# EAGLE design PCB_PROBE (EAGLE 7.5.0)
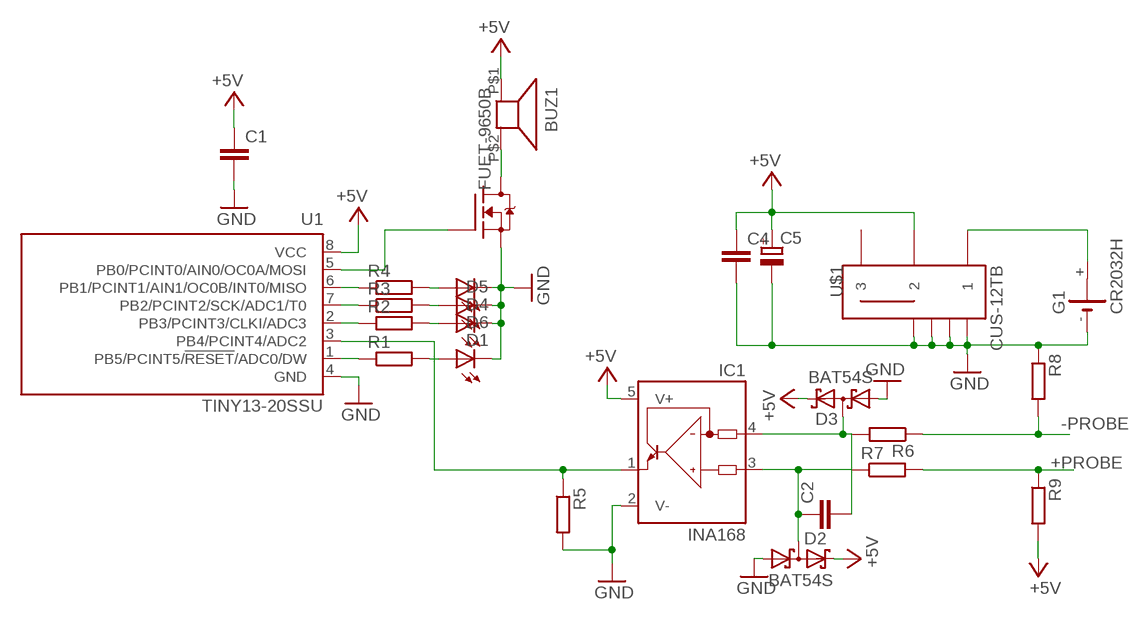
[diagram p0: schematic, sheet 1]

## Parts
BUZ1  FUET-9650B  [FUET-9650B]
C1  C-EUC0603  [C0603]
C2  C-EUC0603  [C0603]
C4  C-EUC0603  [C0603]
C5  CPOL-EUSMCC  [SMC_C]
D1  LEDCHIPLED_0805  [CHIPLED_0805]
D2  BAT54S  [SOT23]
D3  BAT54S  [SOT23]
D4  LEDCHIPLED_0805  [CHIPLED_0805]
D5  LEDCHIPLED_0805  [CHIPLED_0805]
D6  LEDCHIPLED_0805  [CHIPLED_0805]
G1  CR2032H  [CR2032H]
IC1  INA168  [SOT23-5]
Q1  ZVN3310F  [SOT23]
R1  R-EU_R0603  [R0603]
R2  R-EU_R0603  [R0603]
R3  R-EU_R0603  [R0603]
R4  R-EU_R0603  [R0603]
R5  R-EU_R0603  [R0603]
R6  R-EU_R0603  [R0603]
R7  R-EU_R0603  [R0603]
R8  R-EU_R0603  [R0603]
R9  R-EU_R0603  [R0603]
U1  TINY13-20SSU  [8S1]
U$1  CUS-12TB  [CUS-12B]

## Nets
+5V: BUZ1.P$1 C1.1 C4.1 C5.+ D2.2(C2) D3.2(C2) IC1.5(V+) R9.2 U1.8(VCC) U$1.P$2
+PROBE: R7.2 R9.1
-PROBE: R6.1 R8.2
GND: C1.2 C4.2 C5.- D1.C D2.1(A1) D3.1(A1) D4.C D5.C D6.C G1.- IC1.2(V-) Q1.3(S) R5.2 R8.1 U1.4(GND) U$1.P$4(GND) U$1.P$5(GND) U$1.P$6(GND) U$1.P$7(GND)
N$1: G1.+ U$1.P$1
N$2: R1.1 U1.1(PB5/PCINT5/!RESET!/ADC0/DW)
N$3: R2.1 U1.2(PB3/PCINT3/CLKI/ADC3)
N$4: R3.1 U1.7(PB2/PCINT2/SCK/ADC1/T0)
N$5: R4.1 U1.6(PB1/PCINT1/AIN1/OC0B/INT0/MISO)
N$6: D6.A R4.2
N$7: D5.A R3.2
N$8: D4.A R2.2
N$9: D1.A R1.2
N$10: IC1.1(OUT) R5.1 U1.3(PB4/PCINT4/ADC2)
N$11: C2.2 D3.3(C1A2) IC1.4(IN-) R6.2
N$12: C2.1 D2.3(C1A2) IC1.3(IN+) R7.1
N$13: Q1.2(G) U1.5(PB0/PCINT0/AIN0/OC0A/MOSI)
N$14: BUZ1.P$2 Q1.1(D)
Unconnected: G1.+@1(+) U$1.P$3

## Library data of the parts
BUZ1 = buzzer:FUET-9650B
C1 C2 C4 = rcl:C-EU: CAPACITOR, European symbol
C5 = rcl:CPOL-EU: POLARIZED CAPACITOR, European symbol
D1 D4-D6 = led:LED: LED
D2 D3 = diode:BAT54S: Schottky Diodes Pin connection corrected 2011-05-04 Source: Fairchild .. BAT54.pdf
G1 = battery:CR2032H: LI BATTERY Varta
IC1 = burr-brown:INA168: High-Side Measurement Current Shunt Monitor; MF: TEXAS INSTRUMENTS; MPN: INA168NA/250; OC_FARNELL: 4375737; OC_NEWARK: 35C1744
Q1 = transistor-fet:ZVN3310F
R1-R9 = rcl:R-EU_: RESISTOR, European symbol
U1 = atmel:TINY13: 8-bit AVR Microcontroller with 1K Bytes In-System Programmable Flash Source: http://www.atmel.com/dyn/resources/prod_documents/2535S.pdf; MPN: ATTINY13-20SSU; OC_FARNELL: 1455133; OC_NEWARK: 58M3771
U$1 = CUS-12TB:CUS-12TB: Check availability; AVAILABILITY: In Stock; CHECK_PRICES: https://www.snapeda.com/parts/CUS-12TB/Nidec/view-part/?ref=eda; DESCRIPTION: Slide Switch SPDT Surface Mount, Right Angle; MF: Nidec Copal; MP: CUS-12TB; PACKAGE: None; PRICE: None; SNAPEDA_LINK: https://www.snapeda.com/parts/CUS-12TB/Nidec/view-part/?ref=snap

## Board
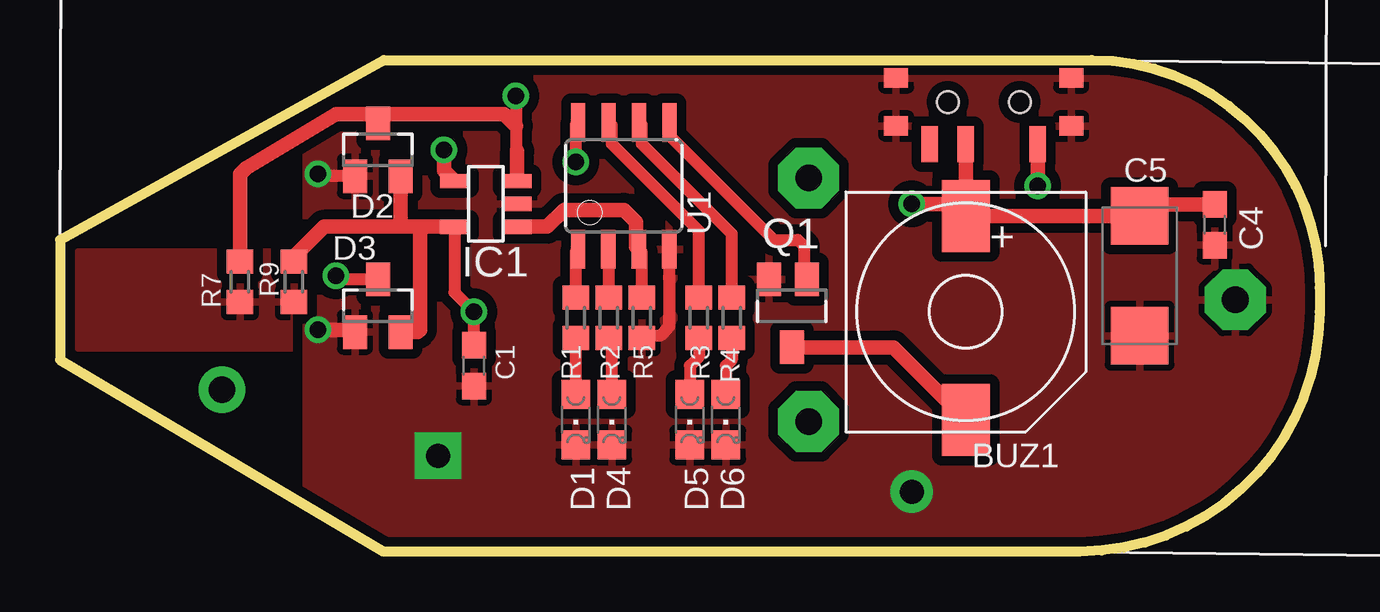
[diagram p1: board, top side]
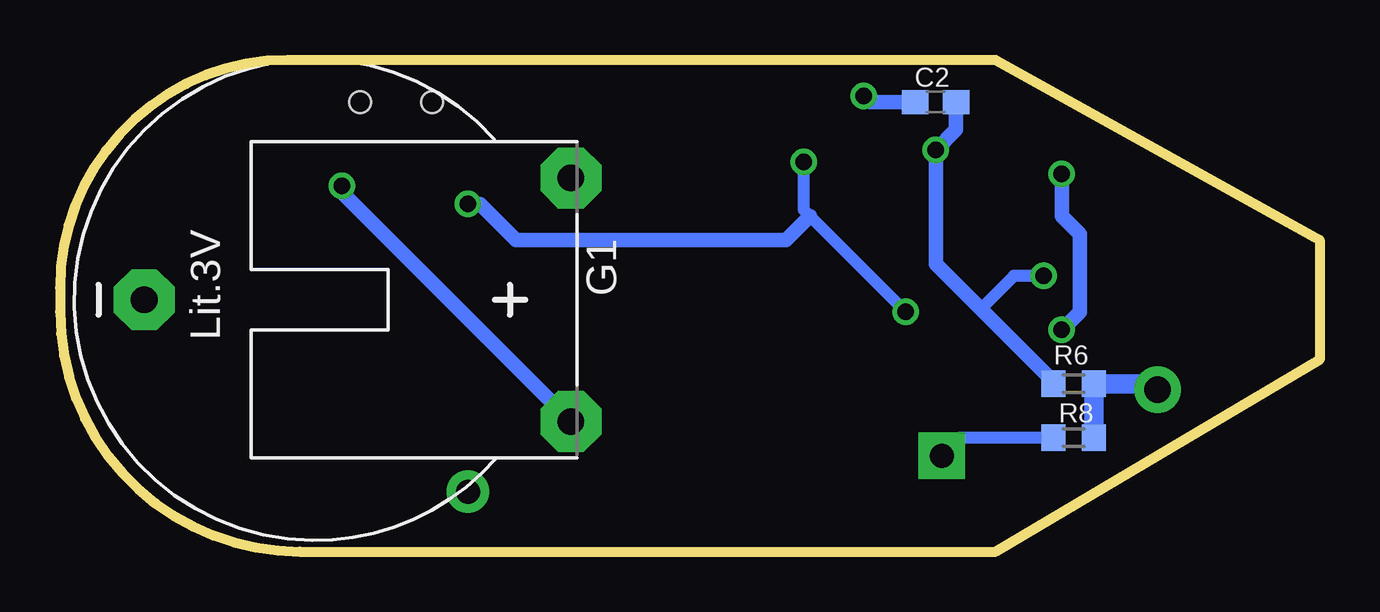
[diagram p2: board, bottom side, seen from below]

Size 52.5 x 20.5 mm. Coordinates in mm from the lower left corner, seen from the top.
Outline: 13.5,20.5 43,20.5 arc-90 52.5,11 52.5,10 arc-90 42.5,0 13.5,0 0,8 0,13 13.5,20.5
Copper layers (1*16): Top 0.035mm / dielectric 1.5mm / Bottom 0.035mm
Design rules "default *": minimum track width 10mil, minimum drill 18mil, track to track 8mil, track to pad 8mil, pad to pad 8mil, via to via 8mil, smd to smd 8mil, copper to edge 5mil, drill to drill 8mil, minimum pad ring 10mil, minimum via ring 8mil, stop-mask expansion 2mil, vias tented up to drill 0mil, thermal gap 10mil
tRestrict: area -44.6,1 to -40.6,2.6

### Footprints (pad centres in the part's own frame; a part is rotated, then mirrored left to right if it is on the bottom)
FUET-9650B = smd 2 x 3: P$1 0,4; P$2 0,-4.5
C0603 = smd 1.1 x 1: 1 -0.85,0; 2 0.85,0
SMC_C = smd 2.4 x 2.4: + -2.5,0; - 2.5,0
CHIPLED_0805 = smd 1.2 x 1.2: A 0,-1.05; C 0,1.05
SOT23 = smd 1 x 1.4: 1 -0.95,-1.1; 2 0.95,-1.1; 3 0,1.1
CR2032H = drill 1.118 pad 2.54 octagon: + 5.08,10.795; +@1 -5.08,10.795; - 0,-6.985
SOT23-5 = smd 0.6 x 1.2: 1 -0.95,-1.306; 2 0,-1.306; 3 0.95,-1.306; 4 0.95,1.306; 5 -0.95,1.306
SOT23' = smd 1 x 1.4: 1 0,1.735; 2 -0.632,-1.1; 3 0.95,-1.1
R0603 = smd 1 x 1.1: 1 -0.85,0; 2 0.85,0
8S1 = smd 0.6 x 1.6: 1 -1.905,-2.654; 2 -0.645,-2.654; 3 0.625,-2.654; 4 1.895,-2.654; 5 1.905,2.654; 6 0.635,2.654; 7 -0.635,2.654; 8 -1.905,2.654
CUS-12B = smd 0.7 x 1.5: P$1 -2.25,1.75; P$2 0.75,1.75; P$3 2.25,1.75 | smd 1 x 0.8: P$4 -3.65,1; P$5 -3.65,-1; P$6 3.65,-1; P$7 3.65,1 | hole 0.9: -1.5,0; 1.5,0

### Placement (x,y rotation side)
BUZ1  37.75,10 0 top
C1  17.25,7.75 270 top
C2  16,18.75 0 bottom
C4  48.12,13.62 270 top
C5  45,11.5 270 top
D1  21.5,5.5 180 top
D2  13.25,16.75 0 top
D3  13.25,10.25 0 top
D4  23,5.5 180 top
D5  26.25,5.5 180 top
D6  27.75,5.5 180 top
G1  42,10.5 270 bottom
IC1  17.75,14.5 90 top
Q1  ZVN3310F  [SOT23']  30.5,10.25 180 top
R1  21.5,9.75 270 top
R2  22.88,9.75 270 top
R3  26.62,9.75 270 top
R4  28,9.75 270 top
R5  24.25,9.75 270 top
R6  10.25,7 180 bottom
R7  7.5,11.25 270 top
R8  10.25,4.75 0 bottom
R9  9.75,11.25 90 top
U1  23.5,15.25 0 top
U$1  38.5,18.75 180 top

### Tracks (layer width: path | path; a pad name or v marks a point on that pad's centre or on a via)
+5V  (via drill 0.7)
  Top 0.5: IC1.5 16.44,10.81 v17.25,10 C1.1 | v21.5,16.25 21.5,17.81 U1.8
  Top 0.61: IC1.5 15,13.55 | 15,13.55 14,13.55 | 14,13.55 11,13.55 9.75,12.3 R9.2 | D2.2 14.2,13.75 14,13.55 | D3.2 14.9,9.15 15,9.25 15,13.55 | C4.1 45.47,14.48 C5.+ BUZ1.P$1 U$1.P$2 37.75,14.5 v35.5,14.5
  Bottom 0.5: v17.25,10 21.25,14 21.5,14.25 v21.5,16.25
  Bottom 0.61: v35.5,14.5 35,14.5 33.5,13 22.25,13 21.25,14
+PROBE
  pour Top (isolate 0.406, rank 2): 0.75,12.5 10.25,12.5 10.25,8.5 0.75,8.5
-PROBE  (via drill 1.1 pad 1.93)
  Bottom 0.813: R8.2 R6.1 7,7 v6.75,6.75
GND  (via drill 0.7, 1 pad 1.78, 1 pad 1.93)
  Top 0.5: U1.4 25.39,9.39 25,9 24.35,9 R5.2 | D2.1 10.85,15.65 v10.75,15.75
  Top 0.61: v10.75,9.25 12.2,9.25 D3.1
  Bottom 0.5: R8.1 15,4.75 v15.75,4
  Bottom 0.61: v10.75,15.75 10.75,14 10,13.25 10,10 v10.75,9.25
  other vias: 35.5,2.5
  pour Top (isolate 0.406): 10.25,20.75 53,20.75 53,-0.5 10.25,-0.5
N$1  (via drill 0.7)
  Top 0.61: U$1.P$1 v40.75,15.25
  Bottom 0.61: v40.75,15.25 40.75,14.96 G1.+
N$2
  Top 0.5: R1.1 21.5,12.5 U1.1
N$3
  Top 0.5: R2.1 22.88,12.58 U1.2
N$4
  Top 0.5: U1.7 23,17.77 23,17 26.62,13.38 R3.1
N$5
  Top 0.5: R4.1 28,13.25 24.25,17 24.25,17.79 U1.6
N$6
  Top 0.5: R4.2 28,8 27.75,7.75 D6.A
N$7
  Top 0.5: R3.2 26.62,8.12 26.25,7.75 D5.A
N$8
  Top 0.5: D4.A 23,8.78 R2.2
N$9
  Top 0.5: D1.A R1.2
N$10
  Top 0.5: R5.1 24.25,12.47 U1.3
  Top 0.61: IC1.1 20.3,13.55 21,14.25 23.5,14.25 24,13.75 24,12.72 U1.3
N$11  (via drill 0.7)
  Top 0.5: D3.3 11.65,11.35 v11.5,11.5
  Top 0.61: v16,16.75 16,15.89 IC1.4
  Bottom 0.5: v11.5,11.5 12.75,11.5 14.12,10.12
  Bottom 0.61: R6.2 11.1,7.1 14.12,10.12 16,12 v16,16.75 15.15,17.6 C2.2
N$12  (via drill 0.7)
  Top 0.5: v19,19 19,17.75 19,16.75 19.06,16.69
  Top 0.61: R7.1 7.5,15.75 7.75,16 11.5,18.25 12.85,18.25 D2.3 13.65,18.25 18.5,18.25 19,17.75 | IC1.3 19.06,16.69
  Bottom 0.61: C2.1 18.75,18.75 v19,19
N$13
  Top 0.5: U1.5 25.41,17.34 29.75,13 30.75,13 31,12.75 31,11.48 Q1.2
N$14
  Top 0.61: Q1.1 34.73,8.52 BUZ1.P$2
